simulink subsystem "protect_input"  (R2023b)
settings: Solver=VariableStepAuto  StartTime=0.0  StopTime=10.0  RelTol=1e-3
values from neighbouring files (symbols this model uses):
  FRE_time_step = 0.005
                
                    
                        1
                        Auto
                        
                        
                        -1.0
                        0
                        Simulink
                        Parameter
                        Default    [run_FRE_data.sldd]
  sim_stop_time = 30.0
                
                    
                        1
                        Auto
                        
                        
                        -1.0
                        0
                        Simulink
                        Parameter
                        Default    [run_FRE_data.sldd]

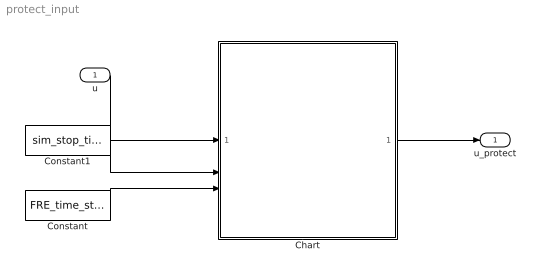
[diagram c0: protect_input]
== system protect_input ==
  u : Inport
  Chart : Stateflow chart  TreatAsAtomicUnit=on
  Constant : Constant  Value=FRE_time_step
  Constant1 : Constant  Value=sim_stop_time
  u_protect : Outport
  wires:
  u/1 -> Chart/1(u)
  Chart/1(u_protect) -> u_protect/1
  Constant1/1 -> Chart/2(tf)
  Constant/1 -> Chart/3(ts)

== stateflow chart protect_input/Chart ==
  state StandBy
    entry:
    u_protect = 0;
    during:
    u_protect = 0;
  state Normal
    entry:
    u_protect = u;
    during:
    u_protect = u;
  state Terminate
    entry:
    u_protect = 0;
    during:
    u_protect = 0;
  (default) -> StandBy
  StandBy -> Normal : [ after(init_time, sec) ]
  Normal -> Terminate : [ after(tf - ts -init_time, sec) ]
  data: u input; u_protect output; init_time parameter; tf input; ts input
